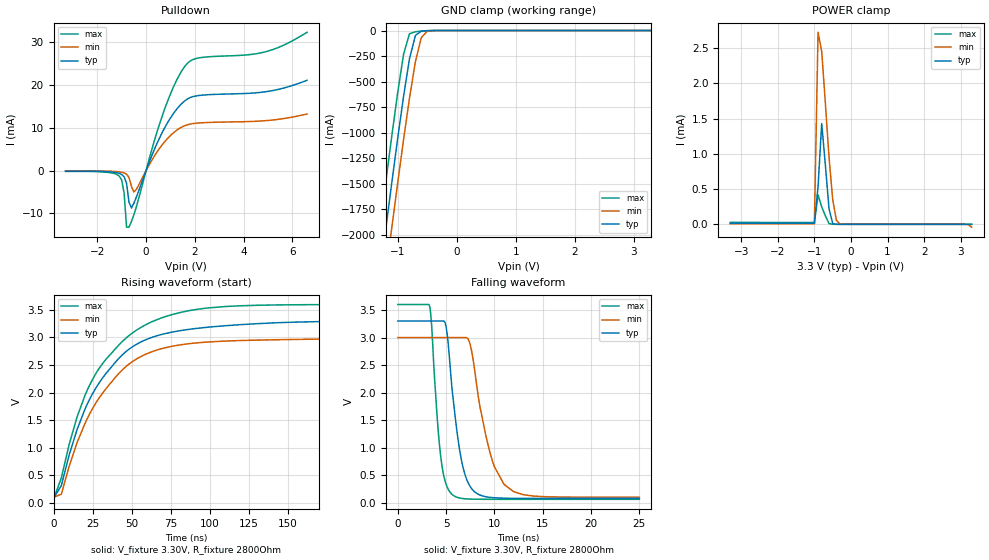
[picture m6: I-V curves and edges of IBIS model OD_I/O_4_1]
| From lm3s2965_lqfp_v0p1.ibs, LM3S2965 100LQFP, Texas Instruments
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[Model]   OD_I/O_4_1
Model_type   I/O_open_drain
Polarity   Inverting
Vinl = 1.26
Vinh = 2.04
Vmeas = 1.65
Rref = 2800
Vref = 3.3
| variable   typ   min   max
C_comp   9.739pF   9.739pF   9.739pF
[Model Spec]
Vinh+   1.91   1.78   2.04
Vinh-   1.90   1.76   2.03
Vinl+   1.40   1.27   1.54
Vinl-   1.39   1.26   1.53
| variable   typ   min   max
[Temperature Range]  25   85   -40
[Voltage Range]   3.3V   3.0V   3.6V
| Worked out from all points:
|   slope of the pulldown table from 0 to 0.495 V, typ, clamps not added: 71.5 ohm
|   GND clamp passes 1 mA (typ) near -0.48 V on its own axis
|   POWER clamp passes 1 mA (typ) near -0.73 V on its own axis
|   falling waveform, V_fixture 3.30V, R_fixture 2800Ohm: 20-80 % time 1.31ns typ, 2ns min, 884ps max; typ from 3.3 V to 0.075 V
|   rising waveform, V_fixture 3.30V, R_fixture 2800Ohm: 20-80 % time 34.2ns typ, 34ns min, 35.2ns max; typ from 0.075 V to 3.3 V
[Pulldown]
|  Voltage   I(typ)   I(min)   I(max)
-3.3V     -128.3uA   -72.81uA   -182.3uA
-1.1V     -636.5uA   -293.8uA   -1.284mA
-900mV    -1.443mA   -530.4uA   -5.27mA
-800mV    -2.996mA   -835.1uA   -13.2mA
-700mV    -7.355mA   -1.607mA   -13.16mA
-600mV    -8.716mA   -3.66mA    -11.87mA
-500mV    -7.628mA   -5mA       -10.33mA
700mV     9.309mA    6.304mA    13.37mA
1.2V      13.92mA    9.18mA     20.46mA
1.7V      16.72mA    10.71mA    25.07mA
4.9V      18.4mA     11.65mA    27.73mA
6.6V      21.07mA    13.21mA    32.27mA
[GND Clamp]
|  Voltage   I(typ)   I(min)   I(max)
-3.3V     -11.72A    -12.12A    -11.3A
-1.4V     -2.845A    -3.285A    -2.387A
-1.3V     -2.39A     -2.831A    -1.93A
-1.2V     -1.938A    -2.38A     -1.478A
-1.1V     -1.494A    -1.934A    -1.036A
-1V       -1.059A    -1.496A    -610.6mA
-900mV    -645mA     -1.069A    -232.9mA
-800mV    -277.1mA   -664.4mA   -31.59mA
-700mV    -48.56mA   -306.6mA   -12.09mA
-600mV    -5.558mA   -70.2mA    -6.272mA
-500mV    -1.167mA   -7.88mA    -2.167mA
3.3V      2.282nA    3.101uA    451.3pA
[POWER Clamp]
|  Voltage   I(typ)   I(min)   I(max)
-3.3V     15.18uA    8.315uA    27.48uA
-1V       14.14uA    7.74uA     25.63uA
-900mV    536uA      2.726mA    416.7uA
-800mV    1.43mA     2.454mA    247.6uA
-700mV    840.7uA    1.719mA    119.9uA
-600mV    221.2uA    951.5uA    11.58uA
-500mV    12.35uA    355.6uA    955.3nA
-400mV    305.2nA    58.59uA    44.3nA
-300mV    9.515nA    3.101uA    1.472nA
3.1V      1.302nA    -112.7nA   143.5pA
3.2V      1.207nA    -2.287uA   131.7pA
3.3V      -104.8pA   -40.34uA   119.2pA
[Ramp]
| variable   typ   min   max
dV/dt_f   1.93/1.31n   1.74/2.00n   2.12/0.88n
dV/dt_r   1.93/34.25n   1.74/33.98n   2.12/35.16n
R_load = 2800Ohm
[Falling Waveform]
V_fixture = 3.30V
V_fixture_min = 3.00V
V_fixture_max = 3.60V
R_fixture = 2800Ohm
|   Time   V(typ)   V(min)   V(max)
0s        3.3V       2.999V     3.6V
3.3ns     3.3V       2.999V     3.562V
4.4ns     3.3V       2.999V     882.5mV
5ns       3.182V     2.999V     326.2mV
5.7ns     1.911V     2.999V     135.1mV
6.5ns     842mV      2.999V     78.99mV
7.3ns     348.3mV    2.963V     64.72mV
9.4ns     97.23mV    999.1mV    59.1mV
11ns      79.28mV    328.4mV    58.76mV
25ns      75.04mV    97.58mV    58.6mV
[Rising Waveform]
V_fixture = 3.30V
V_fixture_min = 3.00V
V_fixture_max = 3.60V
R_fixture = 2800Ohm
|   Time   V(typ)   V(min)   V(max)
0s        74.96mV    97.48mV    58.55mV
5ns       308.3mV    150.6mV    448mV
10ns      863.7mV    661mV      1.057V
15ns      1.321V     1.084V     1.549V
25ns      1.98V      1.709V     2.238V
43ns      2.655V     2.382V     2.898V
60ns      2.97V      2.708V     3.245V
82ns      3.128V     2.869V     3.459V
110ns     3.214V     2.935V     3.562V
250ns     3.298V     2.994V     3.599V
